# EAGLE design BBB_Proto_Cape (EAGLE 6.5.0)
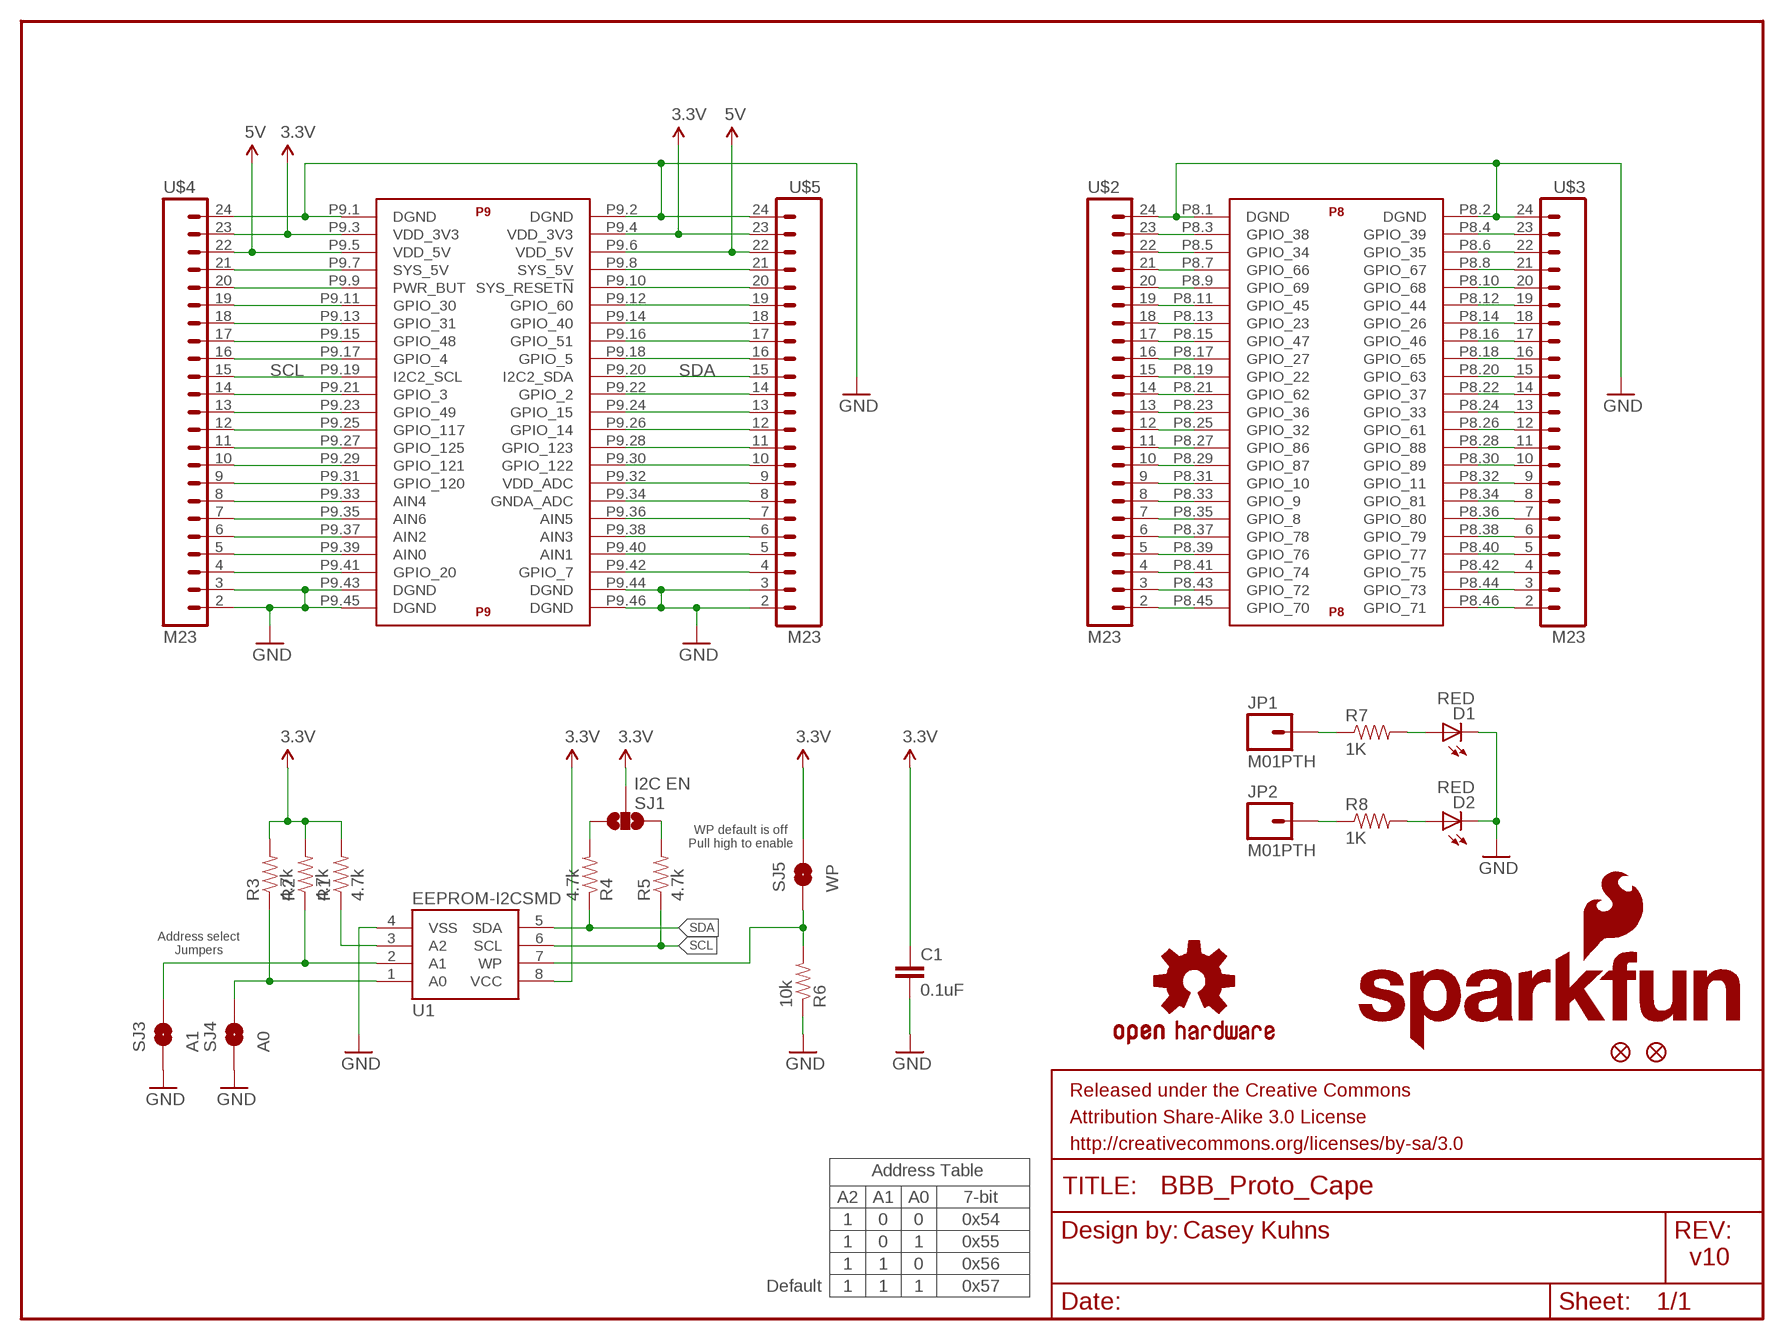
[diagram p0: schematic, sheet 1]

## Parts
C1  0.1uF  0.1UF-25V(+80/-20%)(0603)  [0603-CAP]
D1  RED  LED-RED0603  [LED-0603]
D2  RED  LED-RED0603  [LED-0603]
FID1  FIDUCIAL1X2  [FIDUCIAL-1X2]
FID2  FIDUCIAL1X2  [FIDUCIAL-1X2]
FRAME1  FRAME-LETTER  [CREATIVE_COMMONS]
JP1  M01PTH  [1X01]
JP2  M01PTH  [1X01]
LOGO2  OSHW-LOGOS  [OSHW-LOGO-S]
LOGO3  SFE_LOGO_NAME_FLAME.1_INCH  [SFE_LOGO_NAME_FLAME_.1]
R1  4.7k  4.7KOHM1/10W1%(0603)  [0603]
R2  4.7k  4.7KOHM1/10W1%(0603)  [0603]
R3  4.7k  4.7KOHM1/10W1%(0603)  [0603]
R4  4.7k  4.7KOHM1/10W1%(0603)  [0603]
R5  4.7k  4.7KOHM1/10W1%(0603)  [0603]
R6  10k  10KOHM1/10W1%(0603)0603  [0603-RES]
R7  1K  1KOHM1/10W1%(0603)  [0603-RES]
R8  1K  1KOHM1/10W1%(0603)  [0603-RES]
SJ1  I2C EN  SOLDERJUMPER_2WAYPASTE1&2&3  [SJ_3_PASTE1&2&3]
SJ3  A1  SOLDERJUMPERNO  [SJ_2S-NO]
SJ4  A0  SOLDERJUMPERNO  [SJ_2S-NO]
SJ5  WP  SOLDERJUMPERNO  [SJ_2S-NO]
U1  EEPROM-I2CSMD  [SO08]
U$1  BEAGLE_BONE_BLACK_CAPE  [BEAGLE_BONE_BLACK_CAPE]
U$2  M23  [1X23]
U$3  M23  [1X23]
U$4  M23  [1X23]
U$5  M23  [1X23]

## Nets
3.3V: C1.1 R1.2 R2.2 R3.2 SJ1.2 SJ5.2 U1.8(VCC) U$1.P9.3(P9:VDD_3V3) U$1.P9.4(P9:VDD_3V3) U$4.23 U$5.23
5V: U$1.P9.5(P9:VDD_5V) U$1.P9.6(P9:VDD_5V) U$4.22 U$5.22
A0: R3.1 SJ4.2 U1.1(A0)
A1: R2.1 SJ3.2 U1.2(A1)
GND: C1.2 D1.C D2.C R6.1 SJ3.1 SJ4.1 U1.4(VSS) U$1.P8.1(P8:DGND) U$1.P8.2(P8:DGND) U$1.P9.1(P9:DGND) U$1.P9.2(P9:DGND) U$1.P9.43(P9:DGND) U$1.P9.44(P9:DGND) U$1.P9.45(P9:DGND) U$1.P9.46(P9:DGND) U$2.24 U$3.24 U$4.2 U$4.3 U$4.24 U$5.2 U$5.3 U$5.24
N$1: R6.2 SJ5.1 U1.7(WP)
N$2: U$1.P8.45(P8:GPIO_70) U$2.2
N$3: D1.A R7.2
N$4: U$1.P8.43(P8:GPIO_72) U$2.3
N$5: U$1.P8.41(P8:GPIO_74) U$2.4
N$6: R1.1 U1.3(A2)
N$7: D2.A R8.2
N$8: JP1.1 R7.1
N$9: U$1.P8.39(P8:GPIO_76) U$2.5
N$10: R4.2 SJ1.3
N$11: R5.2 SJ1.1
N$12: U$1.P8.37(P8:GPIO_78) U$2.6
N$13: U$1.P8.35(P8:GPIO_8) U$2.7
N$14: U$1.P8.33(P8:GPIO_9) U$2.8
N$15: U$1.P8.31(P8:GPIO_10) U$2.9
N$16: U$1.P8.29(P8:GPIO_87) U$2.10
N$17: U$1.P8.27(P8:GPIO_86) U$2.11
N$18: U$1.P8.25(P8:GPIO_32) U$2.12
N$19: U$1.P8.23(P8:GPIO_36) U$2.13
N$20: U$1.P8.21(P8:GPIO_62) U$2.14
N$21: U$1.P8.19(P8:GPIO_22) U$2.15
N$22: U$1.P8.17(P8:GPIO_27) U$2.16
N$23: U$1.P8.15(P8:GPIO_47) U$2.17
N$24: U$1.P8.13(P8:GPIO_23) U$2.18
N$25: U$1.P8.11(P8:GPIO_45) U$2.19
N$26: U$1.P8.9(P8:GPIO_69) U$2.20
N$27: U$1.P8.7(P8:GPIO_66) U$2.21
N$28: U$1.P8.5(P8:GPIO_34) U$2.22
N$29: U$1.P8.3(P8:GPIO_38) U$2.23
N$30: JP2.1 R8.1
N$31: U$1.P8.46(P8:GPIO_71) U$3.2
N$32: U$1.P8.44(P8:GPIO_73) U$3.3
N$33: U$1.P8.42(P8:GPIO_75) U$3.4
N$34: U$1.P8.40(P8:GPIO_77) U$3.5
N$35: U$1.P8.38(P8:GPIO_79) U$3.6
N$36: U$1.P8.36(P8:GPIO_80) U$3.7
N$37: U$1.P8.34(P8:GPIO_81) U$3.8
N$38: U$1.P8.32(P8:GPIO_11) U$3.9
N$39: U$1.P8.30(P8:GPIO_89) U$3.10
N$40: U$1.P8.28(P8:GPIO_88) U$3.11
N$41: U$1.P8.26(P8:GPIO_61) U$3.12
N$42: U$1.P8.24(P8:GPIO_33) U$3.13
N$43: U$1.P8.22(P8:GPIO_37) U$3.14
N$44: U$1.P8.20(P8:GPIO_63) U$3.15
N$45: U$1.P8.18(P8:GPIO_65) U$3.16
N$46: U$1.P8.16(P8:GPIO_46) U$3.17
N$47: U$1.P8.14(P8:GPIO_26) U$3.18
N$48: U$1.P8.12(P8:GPIO_44) U$3.19
N$49: U$1.P8.10(P8:GPIO_68) U$3.20
N$50: U$1.P8.8(P8:GPIO_67) U$3.21
N$51: U$1.P8.6(P8:GPIO_35) U$3.22
N$52: U$1.P8.4(P8:GPIO_39) U$3.23
N$56: U$1.P9.42(P9:GPIO_7) U$5.4
N$57: U$1.P9.40(P9:AIN1) U$5.5
N$58: U$1.P9.38(P9:AIN3) U$5.6
N$59: U$1.P9.36(P9:AIN5) U$5.7
N$60: U$1.P9.34(P9:GNDA_ADC) U$5.8
N$61: U$1.P9.32(P9:VDD_ADC) U$5.9
N$62: U$1.P9.30(P9:GPIO_122) U$5.10
N$63: U$1.P9.28(P9:GPIO_123) U$5.11
N$64: U$1.P9.26(P9:GPIO_14) U$5.12
N$65: U$1.P9.24(P9:GPIO_15) U$5.13
N$66: U$1.P9.22(P9:GPIO_2) U$5.14
N$68: U$1.P9.18(P9:GPIO_5) U$5.16
N$69: U$1.P9.16(P9:GPIO_51) U$5.17
N$70: U$1.P9.14(P9:GPIO_40) U$5.18
N$71: U$1.P9.12(P9:GPIO_60) U$5.19
N$72: U$1.P9.10(P9:SYS_RESET!N) U$5.20
N$73: U$1.P9.8(P9:SYS_5V) U$5.21
N$79: U$1.P9.41(P9:GPIO_20) U$4.4
N$80: U$1.P9.39(P9:AIN0) U$4.5
N$81: U$1.P9.37(P9:AIN2) U$4.6
N$82: U$1.P9.35(P9:AIN6) U$4.7
N$83: U$1.P9.33(P9:AIN4) U$4.8
N$84: U$1.P9.31(P9:GPIO_120) U$4.9
N$85: U$1.P9.29(P9:GPIO_121) U$4.10
N$86: U$1.P9.27(P9:GPIO_125) U$4.11
N$87: U$1.P9.25(P9:GPIO_117) U$4.12
N$88: U$1.P9.23(P9:GPIO_49) U$4.13
N$89: U$1.P9.21(P9:GPIO_3) U$4.14
N$91: U$1.P9.17(P9:GPIO_4) U$4.16
N$92: U$1.P9.15(P9:GPIO_48) U$4.17
N$93: U$1.P9.13(P9:GPIO_31) U$4.18
N$94: U$1.P9.11(P9:GPIO_30) U$4.19
N$95: U$1.P9.9(P9:PWR_BUT) U$4.20
N$96: U$1.P9.7(P9:SYS_5V) U$4.21
SCL: R5.1 U1.6(SCL) U$1.P9.19(P9:I2C2_SCL) U$4.15
SDA: R4.1 U1.5(SDA) U$1.P9.20(P9:I2C2_SDA) U$5.15

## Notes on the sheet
- WP default is off
  Pull high to enable
- Address select
  Jumpers
- Address Table
- A2 | A1 | A0 | 7-bit
- 1 | 0 | 0 | 0x54
- Casey Kuhns
- 1 | 0 | 1 | 0x55
- 1 | 1 | 0 | 0x56 | v10
- Default | 1 | 1 | 1 | 0x57

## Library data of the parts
C1 = SparkFun-Capacitors:0.1UF-25V(+80/-20%)(0603): CAP-00810; PROD_ID: CAP-00810
D1 D2 = SparkFun-LED:LED-RED: Assorted Red LEDs; PROD_ID: DIO-00819
FID1 FID2 = SparkFun-Aesthetics:FIDUCIAL: Fiducial Alignment Points
FRAME1 = SparkFun-Aesthetics:FRAME-LETTER: Schematic Frame
JP1 JP2 = SparkFun-Connectors:M01: Header 1
LOGO2 = SparkFun-Aesthetics:OSHW-LOGO: Open Source Hardware Logo This logo indicates the piece of hardware it is found on incorporates a OSHW license and/or adheres to the definition of open source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
LOGO3 = SparkFun-Aesthetics:SFE_LOGO_NAME_FLAME: SFE Logo, name and flame
R1-R5 = SparkFun-Resistors:4.7KOHM1/10W1%(0603): RES-07857; PROD_ID: RES-07857
R6 = SparkFun-Resistors:10KOHM1/10W1%(0603): RES-00824; PROD_ID: RES-00824; VALUE: 10K
R7 R8 = SparkFun-Resistors:1KOHM1/10W1%(0603): RES-07856; PROD_ID: RES-07856
SJ1 = SparkFun-Passives:SOLDERJUMPER_2WAY: Solder Jumper 2 way solder jumper
SJ3-SJ5 = SparkFun-Passives:SOLDERJUMPER: Solder Jumper
U1 = SparkFun-DigitalIC:EEPROM-I2C: I2C EEPROM chips, 24LC256 (and others)
U$1 = SparkFun-Boards:BEAGLE_BONE_BLACK_CAPE
U$2-U$5 = SparkFun-Connectors:M23

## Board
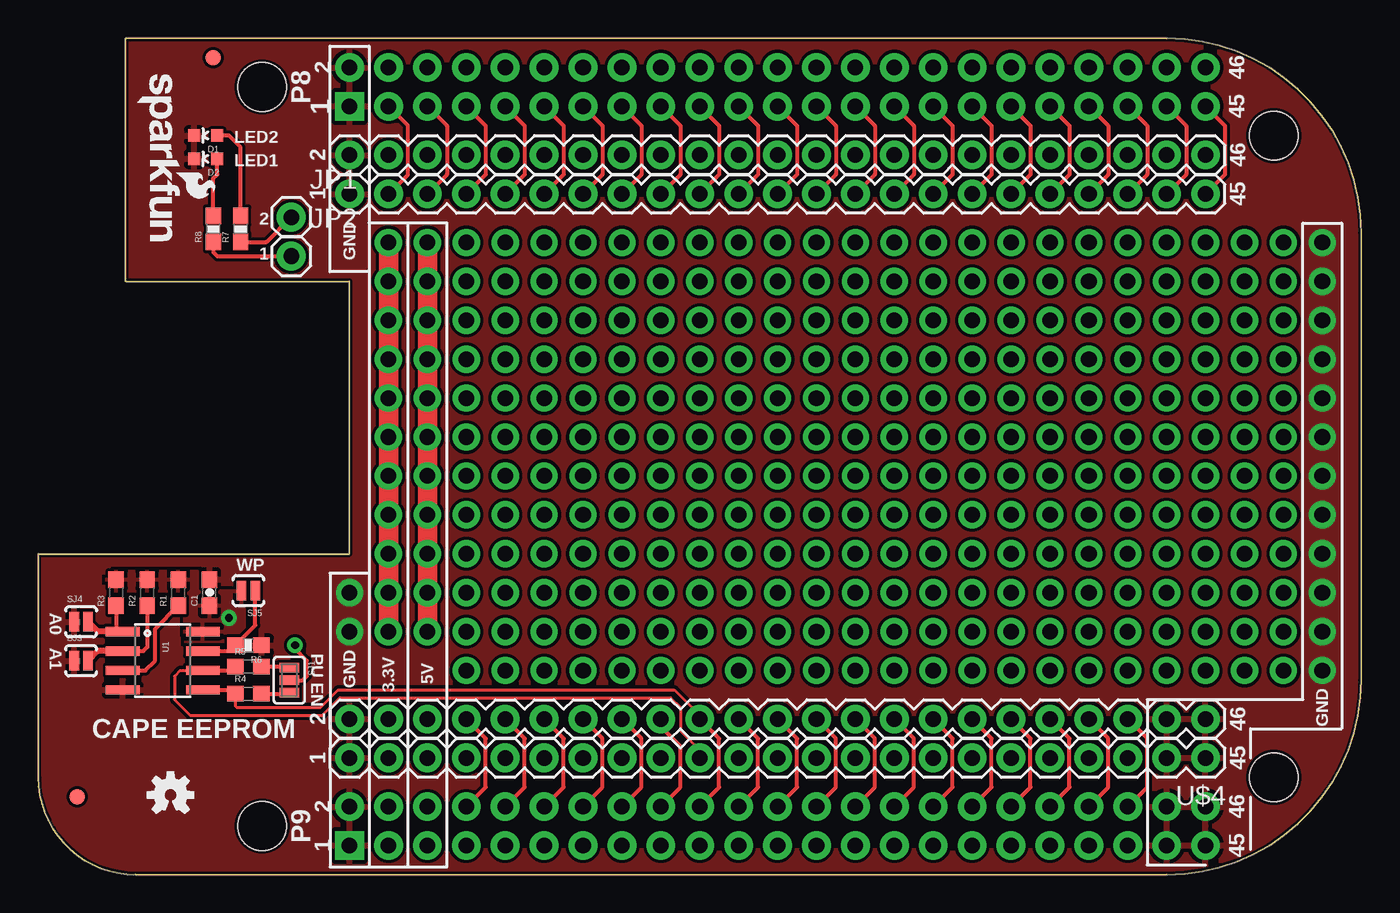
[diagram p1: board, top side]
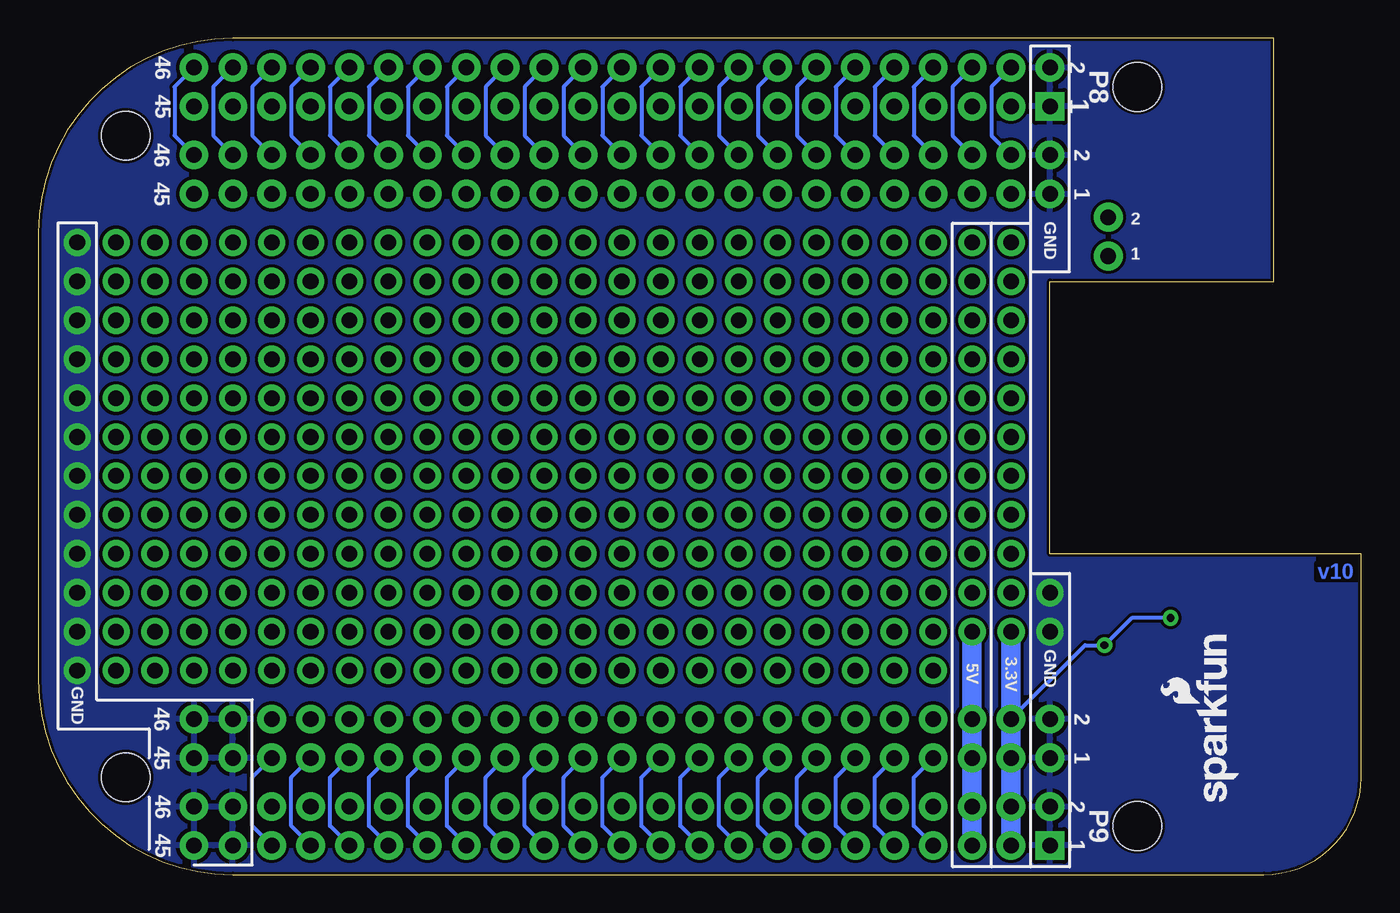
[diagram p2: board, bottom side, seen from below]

Size 86.36 x 54.61 mm. Coordinates in mm from the lower left corner, seen from the top.
Outline: 0,20.95 20.32,20.95 20.32,38.73 5.71,38.73 5.71,54.61 73.66,54.61 arc-90 86.36,41.91 86.36,12.7 arc-90 73.66,0 6.35,0 arc-90 0,6.35 0,20.95
Copper layers (1*16): Top 0.035mm / dielectric 1.5mm / Bottom 0.035mm
Design rules "SparkFun-2-layer": minimum track width 7mil, minimum drill 15mil, track to track 8mil, track to pad 8mil, pad to pad 8mil, via to via 8mil, smd to smd 8mil, copper to edge 8mil, drill to drill 8mil, minimum pad ring 12mil, minimum via ring 10mil, stop-mask expansion 4mil, vias tented up to drill 20mil, thermal gap 10mil

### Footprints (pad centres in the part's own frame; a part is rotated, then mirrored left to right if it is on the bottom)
0603-CAP = smd 1.1 x 1: 1 -0.85,0; 2 0.85,0
LED-0603 = smd 0.8 x 0.8: A 0,-0.75; C 0,0.75
FIDUCIAL-1X2 = smd 1 x 1: 1 0,0
1X01 = drill 1.016 pad 1.88: 1 0,0
0603 = smd 1.1 x 1: 1 -0.85,0; 2 0.85,0
0603-RES = smd 1.1 x 1: 1 -0.85,0; 2 0.85,0
SJ_3_PASTE1&2&3 = smd 0.635 x 1.27: 1 -0.813,0; 2 0,0; 3 0.813,0
SJ_2S-NO = smd 0.635 x 1.27: 1 -0.45,0; 2 0.45,0
SO08 = smd 0.61 x 2.21: 1 -1.905,-2.616; 2 -0.635,-2.616; 3 0.635,-2.616; 4 1.905,-2.616; 5 1.905,2.616; 6 0.635,2.616; 7 -0.635,2.616; 8 -1.905,2.616
BEAGLE_BONE_BLACK_CAPE = drill 1.016 pad 1.88 square: P8.1 20.32,50.165; P9.1 20.32,1.905 | drill 1.016 pad 1.88: P8.2 20.32,52.705; P8.3 22.86,50.165; P8.4 22.86,52.705; P8.5 25.4,50.165; P8.6 25.4,52.705; P8.7 27.94,50.165; P8.8 27.94,52.705; P8.9 30.48,50.165; P8.10 30.48,52.705; P8.11 33.02,50.165; P8.12 33.02,52.705; P8.13 35.56,50.165; P8.14 35.56,52.705; P8.15 38.1,50.165; P8.16 38.1,52.705; P8.17 40.64,50.165; P8.18 40.64,52.705; P8.19 43.18,50.165; P8.20 43.18,52.705; P8.21 45.72,50.165; P8.22 45.72,52.705; P8.23 48.26,50.165; P8.24 48.26,52.705; P8.25 50.8,50.165; P8.26 50.8,52.705; P8.27 53.34,50.165; P8.28 53.34,52.705; P8.29 55.88,50.165; P8.30 55.88,52.705; P8.31 58.42,50.165; P8.32 58.42,52.705; P8.33 60.96,50.165; P8.34 60.96,52.705; P8.35 63.5,50.165; P8.36 63.5,52.705; P8.37 66.04,50.165; P8.38 66.04,52.705; P8.39 68.58,50.165; P8.40 68.58,52.705; P8.41 71.12,50.165; P8.42 71.12,52.705; P8.43 73.66,50.165; P8.44 73.66,52.705; P8.45 76.2,50.165; P8.46 76.2,52.705; P9.2 20.32,4.445; P9.3 22.86,1.905; P9.4 22.86,4.445; P9.5 25.4,1.905; P9.6 25.4,4.445; P9.7 27.94,1.905; P9.8 27.94,4.445; P9.9 30.48,1.905; P9.10 30.48,4.445; P9.11 33.02,1.905; P9.12 33.02,4.445; P9.13 35.56,1.905; P9.14 35.56,4.445; P9.15 38.1,1.905; P9.16 38.1,4.445; P9.17 40.64,1.905; P9.18 40.64,4.445; P9.19 43.18,1.905; P9.20 43.18,4.445; P9.21 45.72,1.905; P9.22 45.72,4.445; P9.23 48.26,1.905; P9.24 48.26,4.445; P9.25 50.8,1.905; P9.26 50.8,4.445; P9.27 53.34,1.905; P9.28 53.34,4.445; P9.29 55.88,1.905; P9.30 55.88,4.445; P9.31 58.42,1.905; P9.32 58.42,4.445; P9.33 60.96,1.905; P9.34 60.96,4.445; P9.35 63.5,1.905; P9.36 63.5,4.445; P9.37 66.04,1.905; P9.38 66.04,4.445; P9.39 68.58,1.905; P9.40 68.58,4.445; P9.41 71.12,1.905; P9.42 71.12,4.445; P9.43 73.66,1.905; P9.44 73.66,4.445; P9.45 76.2,1.905; P9.46 76.2,4.445 | hole 3.175: 14.605,3.175; 80.645,6.35; 80.645,48.26; 14.605,51.435
1X23 = drill 1.016 pad 1.88: 2 -26.67,0; 3 -24.13,0; 4 -21.59,0; 5 -19.05,0; 6 -16.51,0; 7 -13.97,0; 8 -11.43,0; 9 -8.89,0; 10 -6.35,0; 11 -3.81,0; 12 -1.27,0; 13 1.27,0; 14 3.81,0; 15 6.35,0; 16 8.89,0; 17 11.43,0; 18 13.97,0; 19 16.51,0; 20 19.05,0; 21 21.59,0; 22 24.13,0; 23 26.67,0; 24 29.21,0

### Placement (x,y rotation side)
C1  11.18,18.41 90 top
D1  10.92,48.26 90 top
D2  10.92,46.74 90 top
FID1  2.54,5.08 0 top
FID2  11.43,53.34 0 top
FRAME1  not placed on the board
JP1  16.51,42.93 0 top
JP2  16.51,40.39 0 top
LOGO2  8.64,5.21 0 top
LOGO3  6.35,52.7 270 top
R1  9.14,18.41 90 top
R2  7.11,18.41 90 top
R3  5.08,18.41 90 top
R4  13.72,11.81 0 top
R5  13.72,13.59 0 top
R6  13.72,14.99 180 top
R7  13.21,42.16 90 top
R8  11.43,42.16 90 top
SJ1  16.38,12.7 270 top
SJ3  2.79,13.97 0 top
SJ4  2.79,16.51 0 top
SJ5  13.72,18.54 180 top
U1  8.13,13.97 270 top
U$1  0,0 0 top
U$2  49.53,44.45 180 top
U$3  49.53,46.99 180 top
U$4  49.53,7.62 180 top
U$5  49.53,10.16 180 top
U$6  [SFE_LOGO_NAME_FLAME_.1]  7.87,4.32 90 bottom

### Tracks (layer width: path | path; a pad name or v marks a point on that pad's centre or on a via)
3.3V  (via drill 0.51, 1.02 pad 1.78)
  Top 0.254: R1.2 9.48,19.14 | SJ1.2 17.27,12.7 17.53,12.95 17.53,13.97 16.76,14.73 v16.76,14.99
  Top 1.27: v22.86,15.88 v22.86,18.41 v22.86,20.95 v22.86,23.5 v22.86,26.04 v22.86,28.57 v22.86,31.11 v22.86,33.66 v22.86,36.2 v22.86,38.73 v22.86,41.27
  Bottom 0.254: U$5.23 18.03,14.99 v16.76,14.99 14.99,16.76 v12.45,16.76
  Bottom 1.27: U$1.P9.3 U$1.P9.4 U$4.23 U$5.23 v22.86,15.88
  pour Top: 9.53,15.24 13.46,15.24 13.46,18.54 10.41,18.54 10.41,19.81 4.45,19.81 4.45,18.54 9.53,18.54
5V  (via drill 1.02 pad 1.78)
  Top 1.27: v25.4,41.27 v25.4,38.73 v25.4,36.2 v25.4,33.66 v25.4,31.11 v25.4,28.57 v25.4,26.04 v25.4,23.5 v25.4,20.95 v25.4,18.41 v25.4,15.88
  Bottom 1.27: U$1.P9.5 U$1.P9.6 U$4.22 U$5.22 v25.4,15.88
A0
  Top 0.254: R3.1 5.08,15.88 U1.1
  Top 0.406: 5.08,15.88 3.88,15.88 SJ4.2
A1
  Top 0.254: R2.1 7.11,14.86 6.86,14.61 U1.2
  Top 0.406: U1.2 3.88,14.61 SJ3.2
GND  (via drill 1.02 pad 1.78)
  other vias: 83.82,13.34 83.82,15.88 83.82,18.41 83.82,20.95 83.82,23.5 83.82,26.04 83.82,28.57 83.82,31.11 83.82,33.66 83.82,36.2 83.82,38.73 83.82,41.27 20.32,15.88 20.32,18.41
  pour Top (rank 6): 0,20.95 20.32,20.95 20.32,38.73 5.71,38.73 5.71,54.61 73.66,54.61 arc-90 86.36,41.91 86.36,12.7 arc-90 73.66,0 6.35,0 arc-90 0,6.35
  pour Bottom: 0,20.95 20.32,20.95 20.32,38.73 5.71,38.73 5.71,54.61 73.66,54.61 arc-90 86.36,41.91 86.36,12.7 arc-90 73.66,0 6.35,0 arc-90 0,6.35
N$1
  Top 0.254: SJ5.1 14.17,16.29 R6.2 12.48,14.61 U1.7
N$2
  Top 0.254: U$1.P8.45 77.47,48.9 77.47,45.72 U$2.2
N$3
  Top 0.254: R7.2 13.21,47.5 12.45,48.26 D1.A
N$4
  Top 0.254: U$1.P8.43 74.93,48.9 74.93,45.72 U$2.3
N$5
  Top 0.254: U$1.P8.41 72.39,48.9 72.39,45.72 U$2.4
N$6
  Top 0.254: U1.3 6.99,13.34 7.62,13.97 7.62,16.04 R1.1
N$7
  Top 0.254: R8.2 11.43,45.47 11.68,45.72 11.68,46.72 D2.A
N$8
  Top 0.254: R7.1 14.9,41.31 JP1.1
N$9
  Top 0.254: U$1.P8.39 69.85,48.9 69.85,45.72 U$2.5
N$10
  Top 0.254: R4.2 16.31,11.81 SJ1.3
N$11
  Top 0.254: R5.2 16.26,13.59 16.38,13.46 SJ1.1
N$12
  Top 0.254: U$1.P8.37 67.31,48.9 67.31,45.72 U$2.6
N$13
  Top 0.254: U$1.P8.35 64.77,48.9 64.77,45.72 U$2.7
N$14
  Top 0.254: U$1.P8.33 62.23,48.9 62.23,45.72 U$2.8
N$15
  Top 0.254: U$1.P8.31 59.69,48.9 59.69,45.72 U$2.9
N$16
  Top 0.254: U$1.P8.29 57.15,48.9 57.15,45.72 U$2.10
N$17
  Top 0.254: U$1.P8.27 54.61,48.9 54.61,45.72 U$2.11
N$18
  Top 0.254: U$1.P8.25 52.07,48.9 52.07,45.72 U$2.12
N$19
  Top 0.254: U$1.P8.23 49.53,48.9 49.53,45.72 U$2.13
N$20
  Top 0.254: U$1.P8.21 46.99,48.9 46.99,45.72 U$2.14
N$21
  Top 0.254: U$1.P8.19 44.45,48.9 44.45,45.72 U$2.15
N$22
  Top 0.254: U$1.P8.17 41.91,48.9 41.91,45.72 U$2.16
N$23
  Top 0.254: U$1.P8.15 39.37,48.9 39.37,45.72 U$2.17
N$24
  Top 0.254: U$1.P8.13 36.83,48.9 36.83,45.72 U$2.18
N$25
  Top 0.254: U$1.P8.11 34.29,48.9 34.29,45.72 U$2.19
N$26
  Top 0.254: U$1.P8.9 31.75,48.9 31.75,45.72 U$2.20
N$27
  Top 0.254: U$1.P8.7 29.21,48.9 29.21,45.72 U$2.21
N$28
  Top 0.254: U$1.P8.5 26.67,48.9 26.67,45.72 U$2.22
N$29
  Top 0.254: U$2.23 24.13,45.72 24.13,48.9 U$1.P8.3
N$30
  Top 0.254: R8.1 11.43,40.64 11.68,40.39 JP2.1
N$31
  Bottom 0.254: U$1.P8.46 77.47,51.44 77.47,48.26 U$3.2
N$32
  Bottom 0.254: U$1.P8.44 74.93,51.44 74.93,48.26 U$3.3
N$33
  Bottom 0.254: U$1.P8.42 72.39,51.44 72.39,48.26 U$3.4
N$34
  Bottom 0.254: U$1.P8.40 69.85,51.44 69.85,48.26 U$3.5
N$35
  Bottom 0.254: U$1.P8.38 67.31,51.44 67.31,48.26 U$3.6
N$36
  Bottom 0.254: U$1.P8.36 64.77,51.44 64.77,48.26 U$3.7
N$37
  Bottom 0.254: U$1.P8.34 62.23,51.44 62.23,48.26 U$3.8
N$38
  Bottom 0.254: U$1.P8.32 59.69,51.44 59.69,48.26 U$3.9
N$39
  Bottom 0.254: U$1.P8.30 57.15,51.44 57.15,48.26 U$3.10
N$40
  Bottom 0.254: U$1.P8.28 54.61,51.44 54.61,48.26 U$3.11
N$41
  Bottom 0.254: U$1.P8.26 52.07,51.44 52.07,48.26 U$3.12
N$42
  Bottom 0.254: U$1.P8.24 49.53,51.44 49.53,48.26 U$3.13
N$43
  Bottom 0.254: U$1.P8.22 46.99,51.44 46.99,48.26 U$3.14
N$44
  Bottom 0.254: U$1.P8.20 44.45,51.44 44.45,48.26 U$3.15
N$45
  Bottom 0.254: U$1.P8.18 41.91,51.44 41.91,48.26 U$3.16
N$46
  Bottom 0.254: U$1.P8.16 39.37,51.44 39.37,48.26 U$3.17
N$47
  Bottom 0.254: U$1.P8.14 36.83,51.44 36.83,48.26 U$3.18
N$48
  Bottom 0.254: U$1.P8.12 34.29,51.44 34.29,48.26 U$3.19
N$49
  Bottom 0.254: U$1.P8.10 31.75,51.44 31.75,48.26 U$3.20
N$50
  Bottom 0.254: U$1.P8.8 29.21,51.44 29.21,48.26 U$3.21
N$51
  Bottom 0.254: U$1.P8.6 26.67,51.44 26.67,48.26 U$3.22
N$52
  Bottom 0.254: U$1.P8.4 24.13,51.44 24.13,48.26 U$3.23
N$56
  Top 0.254: U$1.P9.42 72.39,5.71 72.39,8.89 U$5.4
N$57
  Top 0.254: U$1.P9.40 69.85,5.71 69.85,8.89 U$5.5
N$58
  Top 0.254: U$1.P9.38 67.31,5.71 67.31,8.89 U$5.6
N$59
  Top 0.254: U$1.P9.36 64.77,5.71 64.77,8.89 U$5.7
N$60
  Top 0.254: U$1.P9.34 62.23,5.71 62.23,8.89 U$5.8
N$61
  Top 0.254: U$1.P9.32 59.69,5.71 59.69,8.89 U$5.9
N$62
  Top 0.254: U$1.P9.30 57.15,5.71 57.15,8.89 U$5.10
N$63
  Top 0.254: U$1.P9.28 54.61,5.71 54.61,8.89 U$5.11
N$64
  Top 0.254: U$1.P9.26 52.07,5.71 52.07,8.89 U$5.12
N$65
  Top 0.254: U$1.P9.24 49.53,5.71 49.53,8.89 U$5.13
N$66
  Top 0.254: U$1.P9.22 46.99,5.71 46.99,8.89 U$5.14
N$68
  Top 0.254: U$1.P9.18 41.91,5.71 41.91,8.38 40.64,9.65 U$5.16
N$69
  Top 0.254: U$1.P9.16 39.37,5.71 39.37,8.89 U$5.17
N$70
  Top 0.254: U$1.P9.14 36.83,5.71 36.83,8.89 U$5.18
N$71
  Top 0.254: U$1.P9.12 34.29,5.71 34.29,8.89 U$5.19
N$72
  Top 0.254: U$1.P9.10 31.75,5.71 31.75,8.89 U$5.20
N$73
  Top 0.254: U$1.P9.8 29.21,5.71 29.21,8.89 U$5.21
N$79
  Bottom 0.254: U$1.P9.41 72.39,3.17 72.39,6.35 U$4.4
N$80
  Bottom 0.254: U$1.P9.39 69.85,3.17 69.85,6.35 U$4.5
N$81
  Bottom 0.254: U$1.P9.37 67.31,3.17 67.31,6.35 U$4.6
N$82
  Bottom 0.254: U$1.P9.35 64.77,3.17 64.77,6.35 U$4.7
N$83
  Bottom 0.254: U$1.P9.33 62.23,3.17 62.23,6.35 U$4.8
N$84
  Bottom 0.254: U$1.P9.31 59.69,3.17 59.69,6.35 U$4.9
N$85
  Bottom 0.254: U$1.P9.29 57.15,3.17 57.15,6.35 U$4.10
N$86
  Bottom 0.254: U$1.P9.27 54.61,3.17 54.61,6.35 U$4.11
N$87
  Bottom 0.254: U$1.P9.25 52.07,3.17 52.07,6.35 U$4.12
N$88
  Bottom 0.254: U$1.P9.23 49.53,3.17 49.53,6.35 U$4.13
N$89
  Bottom 0.254: U$1.P9.21 46.99,3.17 46.99,6.35 U$4.14
N$91
  Bottom 0.254: U$1.P9.17 41.91,3.17 41.91,6.35 U$4.16
N$92
  Bottom 0.254: U$1.P9.15 39.37,3.17 39.37,6.35 U$4.17
N$93
  Bottom 0.254: U$1.P9.13 36.83,3.17 36.83,6.35 U$4.18
N$94
  Bottom 0.254: U$1.P9.11 34.29,3.17 34.29,6.35 U$4.19
N$95
  Bottom 0.254: U$1.P9.9 31.75,3.17 31.75,6.35 U$4.20
N$96
  Bottom 0.254: U$1.P9.7 29.21,3.17 29.21,6.35 U$4.21
N$100  (via drill 1.02 pad 1.78)
  other vias: 76.2,13.34
N$101  (via drill 1.02 pad 1.78)
  other vias: 76.2,15.88
N$102  (via drill 1.02 pad 1.78)
  other vias: 76.2,18.41
N$103  (via drill 1.02 pad 1.78)
  other vias: 76.2,20.95
N$104  (via drill 1.02 pad 1.78)
  other vias: 76.2,23.5
N$105  (via drill 1.02 pad 1.78)
  other vias: 76.2,26.04
N$106  (via drill 1.02 pad 1.78)
  other vias: 76.2,28.57
N$107  (via drill 1.02 pad 1.78)
  other vias: 76.2,31.11
N$108  (via drill 1.02 pad 1.78)
  other vias: 76.2,33.66
N$109  (via drill 1.02 pad 1.78)
  other vias: 76.2,36.2
N$110  (via drill 1.02 pad 1.78)
  other vias: 76.2,38.73
N$111  (via drill 1.02 pad 1.78)
  other vias: 76.2,41.27
N$112  (via drill 1.02 pad 1.78)
  other vias: 73.66,13.34
N$113  (via drill 1.02 pad 1.78)
  other vias: 73.66,15.88
N$114  (via drill 1.02 pad 1.78)
  other vias: 73.66,18.41
N$115  (via drill 1.02 pad 1.78)
  other vias: 73.66,20.95
N$116  (via drill 1.02 pad 1.78)
  other vias: 73.66,23.5
N$117  (via drill 1.02 pad 1.78)
  other vias: 73.66,26.04
N$118  (via drill 1.02 pad 1.78)
  other vias: 73.66,28.57
N$119  (via drill 1.02 pad 1.78)
  other vias: 73.66,31.11
N$120  (via drill 1.02 pad 1.78)
  other vias: 73.66,33.66
N$121  (via drill 1.02 pad 1.78)
  other vias: 73.66,36.2
N$122  (via drill 1.02 pad 1.78)
  other vias: 73.66,38.73
N$123  (via drill 1.02 pad 1.78)
  other vias: 73.66,41.27
N$124  (via drill 1.02 pad 1.78)
  other vias: 71.12,13.34
N$125  (via drill 1.02 pad 1.78)
  other vias: 71.12,15.88
N$126  (via drill 1.02 pad 1.78)
  other vias: 71.12,18.41
N$127  (via drill 1.02 pad 1.78)
  other vias: 71.12,20.95
N$128  (via drill 1.02 pad 1.78)
  other vias: 71.12,23.5
N$129  (via drill 1.02 pad 1.78)
  other vias: 71.12,26.04
N$130  (via drill 1.02 pad 1.78)
  other vias: 71.12,28.57
N$131  (via drill 1.02 pad 1.78)
  other vias: 71.12,31.11
N$132  (via drill 1.02 pad 1.78)
  other vias: 71.12,33.66
N$133  (via drill 1.02 pad 1.78)
  other vias: 71.12,36.2
N$134  (via drill 1.02 pad 1.78)
  other vias: 71.12,38.73
N$135  (via drill 1.02 pad 1.78)
  other vias: 71.12,41.27
N$136  (via drill 1.02 pad 1.78)
  other vias: 68.58,13.34
N$137  (via drill 1.02 pad 1.78)
  other vias: 68.58,15.88
N$138  (via drill 1.02 pad 1.78)
  other vias: 68.58,18.41
N$139  (via drill 1.02 pad 1.78)
  other vias: 68.58,20.95
N$140  (via drill 1.02 pad 1.78)
  other vias: 68.58,23.5
N$141  (via drill 1.02 pad 1.78)
  other vias: 68.58,26.04
N$142  (via drill 1.02 pad 1.78)
  other vias: 68.58,28.57
N$143  (via drill 1.02 pad 1.78)
  other vias: 68.58,31.11
N$144  (via drill 1.02 pad 1.78)
  other vias: 68.58,33.66
N$145  (via drill 1.02 pad 1.78)
  other vias: 68.58,36.2
N$146  (via drill 1.02 pad 1.78)
  other vias: 68.58,38.73
N$147  (via drill 1.02 pad 1.78)
  other vias: 68.58,41.27
N$148  (via drill 1.02 pad 1.78)
  other vias: 66.04,13.34
N$149  (via drill 1.02 pad 1.78)
  other vias: 66.04,15.88
N$150  (via drill 1.02 pad 1.78)
  other vias: 66.04,18.41
N$151  (via drill 1.02 pad 1.78)
  other vias: 66.04,20.95
N$152  (via drill 1.02 pad 1.78)
  other vias: 66.04,23.5
N$153  (via drill 1.02 pad 1.78)
  other vias: 66.04,26.04
N$154  (via drill 1.02 pad 1.78)
  other vias: 66.04,28.57
N$155  (via drill 1.02 pad 1.78)
  other vias: 66.04,31.11
N$156  (via drill 1.02 pad 1.78)
  other vias: 66.04,33.66
N$157  (via drill 1.02 pad 1.78)
  other vias: 66.04,36.2
N$158  (via drill 1.02 pad 1.78)
  other vias: 66.04,38.73
N$159  (via drill 1.02 pad 1.78)
  other vias: 66.04,41.27
N$160  (via drill 1.02 pad 1.78)
  other vias: 63.5,13.34
N$161  (via drill 1.02 pad 1.78)
  other vias: 63.5,15.88
N$162  (via drill 1.02 pad 1.78)
  other vias: 63.5,18.41
N$163  (via drill 1.02 pad 1.78)
  other vias: 63.5,20.95
N$164  (via drill 1.02 pad 1.78)
  other vias: 63.5,23.5
N$165  (via drill 1.02 pad 1.78)
  other vias: 63.5,26.04
N$166  (via drill 1.02 pad 1.78)
  other vias: 63.5,28.57
N$167  (via drill 1.02 pad 1.78)
  other vias: 63.5,31.11
N$168  (via drill 1.02 pad 1.78)
  other vias: 63.5,33.66
N$169  (via drill 1.02 pad 1.78)
  other vias: 63.5,36.2
N$170  (via drill 1.02 pad 1.78)
  other vias: 63.5,38.73
N$171  (via drill 1.02 pad 1.78)
  other vias: 63.5,41.27
N$172  (via drill 1.02 pad 1.78)
  other vias: 60.96,13.34
N$173  (via drill 1.02 pad 1.78)
  other vias: 60.96,15.88
N$174  (via drill 1.02 pad 1.78)
  other vias: 60.96,18.41
N$175  (via drill 1.02 pad 1.78)
  other vias: 60.96,20.95
N$176  (via drill 1.02 pad 1.78)
  other vias: 60.96,23.5
N$177  (via drill 1.02 pad 1.78)
  other vias: 60.96,26.04
N$178  (via drill 1.02 pad 1.78)
  other vias: 60.96,28.57
N$179  (via drill 1.02 pad 1.78)
  other vias: 60.96,31.11
N$180  (via drill 1.02 pad 1.78)
  other vias: 60.96,33.66
N$181  (via drill 1.02 pad 1.78)
  other vias: 60.96,36.2
N$182  (via drill 1.02 pad 1.78)
  other vias: 60.96,38.73
N$183  (via drill 1.02 pad 1.78)
  other vias: 60.96,41.27
N$184  (via drill 1.02 pad 1.78)
  other vias: 58.42,13.34
N$185  (via drill 1.02 pad 1.78)
  other vias: 58.42,15.88
N$186  (via drill 1.02 pad 1.78)
  other vias: 58.42,18.41
N$187  (via drill 1.02 pad 1.78)
  other vias: 58.42,20.95
N$188  (via drill 1.02 pad 1.78)
  other vias: 58.42,23.5
N$189  (via drill 1.02 pad 1.78)
  other vias: 58.42,26.04
N$190  (via drill 1.02 pad 1.78)
  other vias: 58.42,28.57
N$191  (via drill 1.02 pad 1.78)
  other vias: 58.42,31.11
N$192  (via drill 1.02 pad 1.78)
  other vias: 58.42,33.66
N$193  (via drill 1.02 pad 1.78)
  other vias: 58.42,36.2
N$194  (via drill 1.02 pad 1.78)
  other vias: 58.42,38.73
N$195  (via drill 1.02 pad 1.78)
  other vias: 58.42,41.27
N$196  (via drill 1.02 pad 1.78)
  other vias: 55.88,13.34
N$197  (via drill 1.02 pad 1.78)
  other vias: 55.88,15.88
N$198  (via drill 1.02 pad 1.78)
  other vias: 55.88,18.41
N$199  (via drill 1.02 pad 1.78)
  other vias: 55.88,20.95
N$200  (via drill 1.02 pad 1.78)
  other vias: 55.88,23.5
N$201  (via drill 1.02 pad 1.78)
  other vias: 55.88,26.04
N$202  (via drill 1.02 pad 1.78)
  other vias: 55.88,28.57
N$203  (via drill 1.02 pad 1.78)
  other vias: 55.88,31.11
N$204  (via drill 1.02 pad 1.78)
  other vias: 55.88,33.66
N$205  (via drill 1.02 pad 1.78)
  other vias: 55.88,36.2
N$206  (via drill 1.02 pad 1.78)
  other vias: 55.88,38.73
N$207  (via drill 1.02 pad 1.78)
  other vias: 55.88,41.27
N$208  (via drill 1.02 pad 1.78)
  other vias: 53.34,13.34
N$209  (via drill 1.02 pad 1.78)
  other vias: 53.34,15.88
N$210  (via drill 1.02 pad 1.78)
  other vias: 53.34,18.41
N$211  (via drill 1.02 pad 1.78)
  other vias: 53.34,20.95
N$212  (via drill 1.02 pad 1.78)
  other vias: 53.34,23.5
N$213  (via drill 1.02 pad 1.78)
  other vias: 53.34,26.04
N$214  (via drill 1.02 pad 1.78)
  other vias: 53.34,28.57
N$215  (via drill 1.02 pad 1.78)
  other vias: 53.34,31.11
N$216  (via drill 1.02 pad 1.78)
  other vias: 53.34,33.66
N$217  (via drill 1.02 pad 1.78)
  other vias: 53.34,36.2
N$218  (via drill 1.02 pad 1.78)
  other vias: 53.34,38.73
N$219  (via drill 1.02 pad 1.78)
  other vias: 53.34,41.27
N$220  (via drill 1.02 pad 1.78)
  other vias: 50.8,13.34
N$221  (via drill 1.02 pad 1.78)
  other vias: 50.8,15.88
N$222  (via drill 1.02 pad 1.78)
  other vias: 50.8,18.41
N$223  (via drill 1.02 pad 1.78)
  other vias: 50.8,20.95
N$224  (via drill 1.02 pad 1.78)
  other vias: 50.8,23.5
N$225  (via drill 1.02 pad 1.78)
  other vias: 50.8,26.04
N$226  (via drill 1.02 pad 1.78)
  other vias: 50.8,28.57
N$227  (via drill 1.02 pad 1.78)
  other vias: 50.8,31.11
N$228  (via drill 1.02 pad 1.78)
  other vias: 50.8,33.66
N$229  (via drill 1.02 pad 1.78)
  other vias: 50.8,36.2
N$230  (via drill 1.02 pad 1.78)
  other vias: 50.8,38.73
N$231  (via drill 1.02 pad 1.78)
  other vias: 50.8,41.27
N$232  (via drill 1.02 pad 1.78)
  other vias: 48.26,13.34
N$233  (via drill 1.02 pad 1.78)
  other vias: 48.26,15.88
N$234  (via drill 1.02 pad 1.78)
  other vias: 48.26,18.41
N$235  (via drill 1.02 pad 1.78)
  other vias: 48.26,20.95
N$236  (via drill 1.02 pad 1.78)
  other vias: 48.26,23.5
N$237  (via drill 1.02 pad 1.78)
  other vias: 48.26,26.04
N$238  (via drill 1.02 pad 1.78)
  other vias: 48.26,28.57
N$239  (via drill 1.02 pad 1.78)
  other vias: 48.26,31.11
N$240  (via drill 1.02 pad 1.78)
  other vias: 48.26,33.66
N$241  (via drill 1.02 pad 1.78)
  other vias: 48.26,36.2
N$242  (via drill 1.02 pad 1.78)
  other vias: 48.26,38.73
N$243  (via drill 1.02 pad 1.78)
  other vias: 48.26,41.27
N$244  (via drill 1.02 pad 1.78)
  other vias: 45.72,13.34
N$245  (via drill 1.02 pad 1.78)
  other vias: 45.72,15.88
N$246  (via drill 1.02 pad 1.78)
  other vias: 45.72,18.41
N$247  (via drill 1.02 pad 1.78)
  other vias: 45.72,20.95
N$248  (via drill 1.02 pad 1.78)
  other vias: 45.72,23.5
N$249  (via drill 1.02 pad 1.78)
  other vias: 45.72,26.04
N$250  (via drill 1.02 pad 1.78)
  other vias: 45.72,28.57
N$251  (via drill 1.02 pad 1.78)
  other vias: 45.72,31.11
N$252  (via drill 1.02 pad 1.78)
  other vias: 45.72,33.66
N$253  (via drill 1.02 pad 1.78)
  other vias: 45.72,36.2
N$254  (via drill 1.02 pad 1.78)
  other vias: 45.72,38.73
N$255  (via drill 1.02 pad 1.78)
  other vias: 45.72,41.27
N$256  (via drill 1.02 pad 1.78)
  other vias: 43.18,13.34
N$257  (via drill 1.02 pad 1.78)
  other vias: 43.18,15.88
N$258  (via drill 1.02 pad 1.78)
  other vias: 43.18,18.41
N$259  (via drill 1.02 pad 1.78)
  other vias: 43.18,20.95
N$260  (via drill 1.02 pad 1.78)
  other vias: 43.18,23.5
N$261  (via drill 1.02 pad 1.78)
  other vias: 43.18,26.04
N$262  (via drill 1.02 pad 1.78)
  other vias: 43.18,28.57
N$263  (via drill 1.02 pad 1.78)
  other vias: 43.18,31.11
N$264  (via drill 1.02 pad 1.78)
  other vias: 43.18,33.66
N$265  (via drill 1.02 pad 1.78)
  other vias: 43.18,36.2
N$266  (via drill 1.02 pad 1.78)
  other vias: 43.18,38.73
N$267  (via drill 1.02 pad 1.78)
  other vias: 43.18,41.27
N$268  (via drill 1.02 pad 1.78)
  other vias: 40.64,13.34
N$269  (via drill 1.02 pad 1.78)
  other vias: 40.64,15.88
N$270  (via drill 1.02 pad 1.78)
  other vias: 40.64,18.41
N$271  (via drill 1.02 pad 1.78)
  other vias: 40.64,20.95
N$272  (via drill 1.02 pad 1.78)
  other vias: 40.64,23.5
N$273  (via drill 1.02 pad 1.78)
  other vias: 40.64,26.04
N$274  (via drill 1.02 pad 1.78)
  other vias: 40.64,28.57
N$275  (via drill 1.02 pad 1.78)
  other vias: 40.64,31.11
N$276  (via drill 1.02 pad 1.78)
  other vias: 40.64,33.66
N$277  (via drill 1.02 pad 1.78)
  other vias: 40.64,36.2
N$278  (via drill 1.02 pad 1.78)
  other vias: 40.64,38.73
N$279  (via drill 1.02 pad 1.78)
  other vias: 40.64,41.27
N$280  (via drill 1.02 pad 1.78)
  other vias: 38.1,13.34
N$281  (via drill 1.02 pad 1.78)
  other vias: 38.1,15.88
N$282  (via drill 1.02 pad 1.78)
  other vias: 38.1,18.41
N$283  (via drill 1.02 pad 1.78)
  other vias: 38.1,20.95
N$284  (via drill 1.02 pad 1.78)
  other vias: 38.1,23.5
N$285  (via drill 1.02 pad 1.78)
  other vias: 38.1,26.04
N$286  (via drill 1.02 pad 1.78)
  other vias: 38.1,28.57
N$287  (via drill 1.02 pad 1.78)
  other vias: 38.1,31.11
N$288  (via drill 1.02 pad 1.78)
  other vias: 38.1,33.66
N$289  (via drill 1.02 pad 1.78)
  other vias: 38.1,36.2
N$290  (via drill 1.02 pad 1.78)
  other vias: 38.1,38.73
N$291  (via drill 1.02 pad 1.78)
  other vias: 38.1,41.27
N$292  (via drill 1.02 pad 1.78)
  other vias: 35.56,13.34
N$293  (via drill 1.02 pad 1.78)
  other vias: 35.56,15.88
N$294  (via drill 1.02 pad 1.78)
  other vias: 35.56,18.41
N$295  (via drill 1.02 pad 1.78)
  other vias: 35.56,20.95
N$296  (via drill 1.02 pad 1.78)
  other vias: 35.56,23.5
N$297  (via drill 1.02 pad 1.78)
  other vias: 35.56,26.04
N$298  (via drill 1.02 pad 1.78)
  other vias: 35.56,28.57
N$299  (via drill 1.02 pad 1.78)
  other vias: 35.56,31.11
N$300  (via drill 1.02 pad 1.78)
  other vias: 35.56,33.66
N$301  (via drill 1.02 pad 1.78)
  other vias: 35.56,36.2
N$302  (via drill 1.02 pad 1.78)
  other vias: 35.56,38.73
N$303  (via drill 1.02 pad 1.78)
  other vias: 35.56,41.27
N$304  (via drill 1.02 pad 1.78)
  other vias: 33.02,13.34
N$305  (via drill 1.02 pad 1.78)
  other vias: 33.02,15.88
N$306  (via drill 1.02 pad 1.78)
  other vias: 33.02,18.41
N$307  (via drill 1.02 pad 1.78)
  other vias: 33.02,20.95
N$308  (via drill 1.02 pad 1.78)
  other vias: 33.02,23.5
N$309  (via drill 1.02 pad 1.78)
  other vias: 33.02,26.04
N$310  (via drill 1.02 pad 1.78)
  other vias: 33.02,28.57
N$311  (via drill 1.02 pad 1.78)
  other vias: 33.02,31.11
N$312  (via drill 1.02 pad 1.78)
  other vias: 33.02,33.66
N$313  (via drill 1.02 pad 1.78)
  other vias: 33.02,36.2
N$314  (via drill 1.02 pad 1.78)
  other vias: 33.02,38.73
N$315  (via drill 1.02 pad 1.78)
  other vias: 33.02,41.27
N$316  (via drill 1.02 pad 1.78)
  other vias: 30.48,13.34
N$317  (via drill 1.02 pad 1.78)
  other vias: 30.48,15.88
N$318  (via drill 1.02 pad 1.78)
  other vias: 30.48,18.41
N$319  (via drill 1.02 pad 1.78)
  other vias: 30.48,20.95
N$320  (via drill 1.02 pad 1.78)
  other vias: 30.48,23.5
N$321  (via drill 1.02 pad 1.78)
  other vias: 30.48,26.04
N$322  (via drill 1.02 pad 1.78)
  other vias: 30.48,28.57
N$323  (via drill 1.02 pad 1.78)
  other vias: 30.48,31.11
N$324  (via drill 1.02 pad 1.78)
  other vias: 30.48,33.66
N$325  (via drill 1.02 pad 1.78)
  other vias: 30.48,36.2
N$326  (via drill 1.02 pad 1.78)
  other vias: 30.48,38.73
N$327  (via drill 1.02 pad 1.78)
  other vias: 30.48,41.27
N$328  (via drill 1.02 pad 1.78)
  other vias: 27.94,13.34
N$329  (via drill 1.02 pad 1.78)
  other vias: 27.94,15.88
N$330  (via drill 1.02 pad 1.78)
  other vias: 27.94,18.41
N$331  (via drill 1.02 pad 1.78)
  other vias: 27.94,20.95
N$332  (via drill 1.02 pad 1.78)
  other vias: 27.94,23.5
N$333  (via drill 1.02 pad 1.78)
  other vias: 27.94,26.04
N$334  (via drill 1.02 pad 1.78)
  other vias: 27.94,28.57
N$335  (via drill 1.02 pad 1.78)
  other vias: 27.94,31.11
N$336  (via drill 1.02 pad 1.78)
  other vias: 27.94,33.66
N$337  (via drill 1.02 pad 1.78)
  other vias: 27.94,36.2
N$338  (via drill 1.02 pad 1.78)
  other vias: 27.94,38.73
N$339  (via drill 1.02 pad 1.78)
  other vias: 27.94,41.27
N$364  (via drill 1.02 pad 1.78)
  other vias: 78.74,41.27
N$365  (via drill 1.02 pad 1.78)
  other vias: 78.74,38.73
N$366  (via drill 1.02 pad 1.78)
  other vias: 78.74,36.2
N$367  (via drill 1.02 pad 1.78)
  other vias: 81.28,38.73
N$368  (via drill 1.02 pad 1.78)
  other vias: 81.28,36.2
N$369  (via drill 1.02 pad 1.78)
  other vias: 78.74,33.66
N$370  (via drill 1.02 pad 1.78)
  other vias: 81.28,33.66
N$371  (via drill 1.02 pad 1.78)
  other vias: 81.28,31.11
N$372  (via drill 1.02 pad 1.78)
  other vias: 78.74,31.11
N$373  (via drill 1.02 pad 1.78)
  other vias: 78.74,28.57
N$374  (via drill 1.02 pad 1.78)
  other vias: 81.28,28.57
N$375  (via drill 1.02 pad 1.78)
  other vias: 81.28,26.04
N$376  (via drill 1.02 pad 1.78)
  other vias: 78.74,26.04
N$377  (via drill 1.02 pad 1.78)
  other vias: 78.74,23.5
N$378  (via drill 1.02 pad 1.78)
  other vias: 78.74,20.95
N$379  (via drill 1.02 pad 1.78)
  other vias: 78.74,18.41
N$380  (via drill 1.02 pad 1.78)
  other vias: 78.74,15.88
N$381  (via drill 1.02 pad 1.78)
  other vias: 81.28,15.88
N$382  (via drill 1.02 pad 1.78)
  other vias: 81.28,18.41
N$383  (via drill 1.02 pad 1.78)
  other vias: 81.28,23.5
N$384  (via drill 1.02 pad 1.78)
  other vias: 81.28,20.95
N$385  (via drill 1.02 pad 1.78)
  other vias: 78.74,13.34
N$386  (via drill 1.02 pad 1.78)
  other vias: 81.28,13.34
N$391  (via drill 1.02 pad 1.78)
  other vias: 81.28,41.27
SCL
  Top 0.203: U1.6 9.27,13.34 8.89,12.95 8.89,11.43 9.91,10.41 18.54,10.41 19.68,11.56 41.27,11.56 41.91,10.92 41.91,9.4 43.18,8.13 U$4.15
  Top 0.254: U1.6 12.61,13.34 R5.1
  Bottom 0.254: U$1.P9.19 44.45,3.17 44.45,6.35 U$4.15
SDA
  Top 0.203: R4.1 12.87,11.01 12.95,10.92 18.41,10.92 19.56,12.06 41.53,12.06 43.18,10.41 U$5.15
  Top 0.254: U1.5 12.61,12.06 R4.1 | U$1.P9.20 44.45,5.71 44.45,8.89 U$5.15

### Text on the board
Bottom: v10
tPlace: LED2 | 2 | 46 | LED1 | 1 | 45 | 2 | 1 | GND | WP | A0 | A1 | PU EN | GND | 3.3V | 5V | GND | CAPE EEPROM | 2 | 46 | 1 | 45
bPlace: 2 | 46 | 1 | 45 | 2 | 1 | GND | GND | 3.3V | 5V | 2 | 46 | GND | 1 | 45
tDocu: Casey Kuhns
